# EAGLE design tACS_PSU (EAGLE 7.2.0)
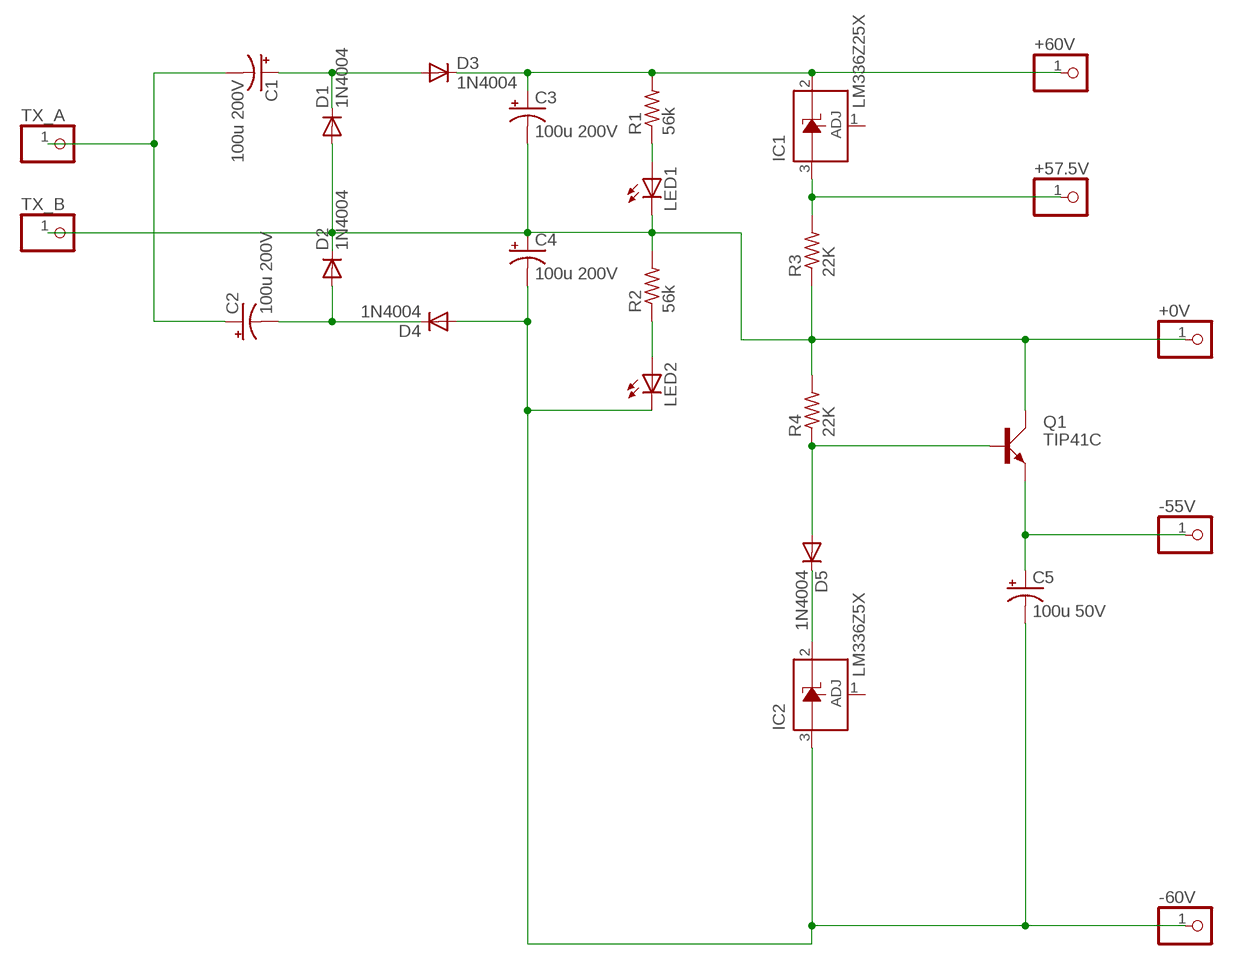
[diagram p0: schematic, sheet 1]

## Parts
+0V  PINHD-1X1  [1X01]
+57.5V  PINHD-1X1  [1X01]
+60V  PINHD-1X1  [1X01]
-55V  PINHD-1X1  [1X01]
-60V  PINHD-1X1  [1X01]
C1  100u 200V  CPOL-USE7.5-18  [E7,5-18]
C2  100u 200V  CPOL-USE7.5-18  [E7,5-18]
C3  100u 200V  CPOL-USE7.5-18  [E7,5-18]
C4  100u 200V  CPOL-USE7.5-18  [E7,5-18]
C5  100u 50V  CPOL-USE3.5-10  [E3,5-10]
D1  1N4004  [DO41-10]
D2  1N4004  [DO41-10]
D3  1N4004  [DO41-10]
D4  1N4004  [DO41-10]
D5  1N4004  [DO41-10]
IC1  LM336Z25X  LM336LP  [TO92]
IC2  LM336Z5X  LM336LP  [TO92]
LED1  LED5MM  [LED5MM]
LED2  LED5MM  [LED5MM]
Q1  TIP41C  [TO220AV]
R1  56k  R-US_0207/10  [0207/10]
R2  56k  R-US_0207/10  [0207/10]
R3  22K  R-US_0207/10  [0207/10]
R4  22K  R-US_0207/10  [0207/10]
TX_A  PINHD-1X1  [1X01]
TX_B  PINHD-1X1  [1X01]

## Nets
N$1: C1.- C2.+ TX_A.1
N$2: +0V.1 C3.- C4.+ D1.A D2.C LED1.K(C) Q1.C R2.2 R3.1 R4.2 TX_B.1
N$3: C2.- D2.A D4.C
N$4: C1.+ D1.C D3.A
N$5: +60V.1 C3.+ D3.C IC1.2(C) R1.2
N$6: -55V.1 C5.+ Q1.E
N$7: -60V.1 C4.- C5.- D4.A IC2.3(A) LED2.K(C)
N$8: LED1.A R1.1
N$10: LED2.A R2.1
N$11: +57.5V.1 IC1.3(A) R3.2
N$12: D5.A Q1.B R4.1
N$13: D5.C IC2.2(C)
Unconnected: IC1.1(ADJ) IC2.1(ADJ)

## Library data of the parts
+0V +57.5V +60V -55V -60V TX_A TX_B = pinhead:PINHD-1X1: PIN HEADER
C1-C5 = rcl:CPOL-US: POLARIZED CAPACITOR, American symbol
D1-D5 = diode:1N4004: DIODE
IC1 IC2 = linear:LM336: 2.5-V INTEGRATED REFERENCE CIRCUITS LM236 Source: http://focus.ti.com/lit/ds/symlink/lm336-2.5.pdf
LED1 LED2 = led:LED: LED
Q1 = transistor-power:TIP41C: NPN TRANSISTOR
R1-R4 = rcl:R-US_: RESISTOR, American symbol

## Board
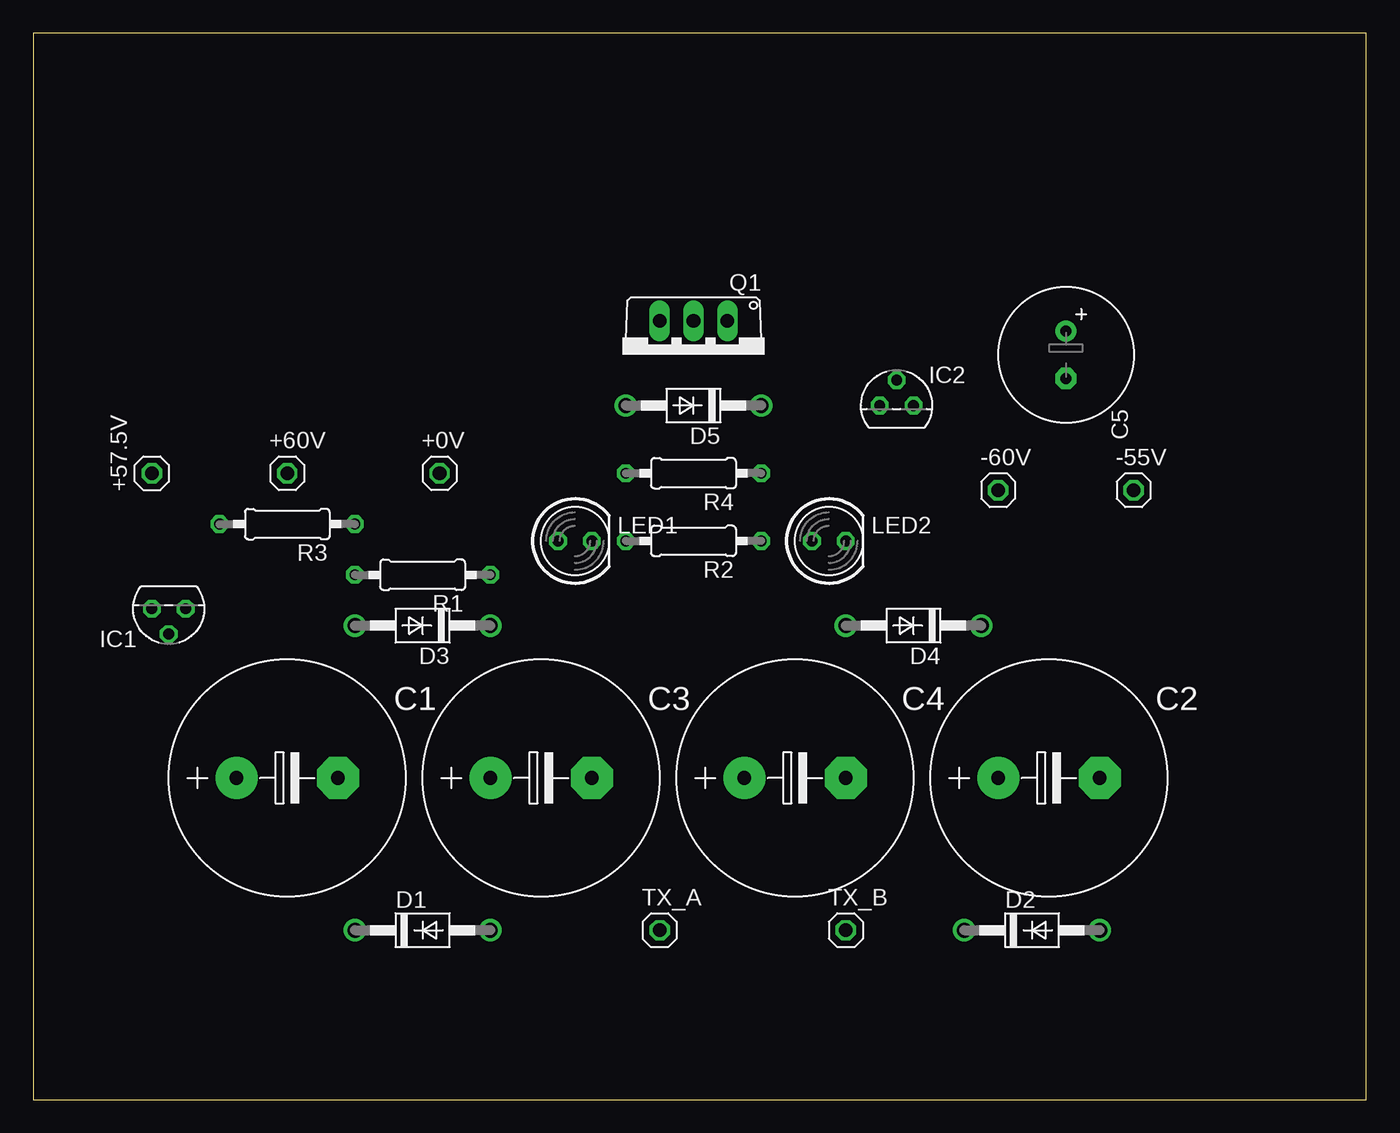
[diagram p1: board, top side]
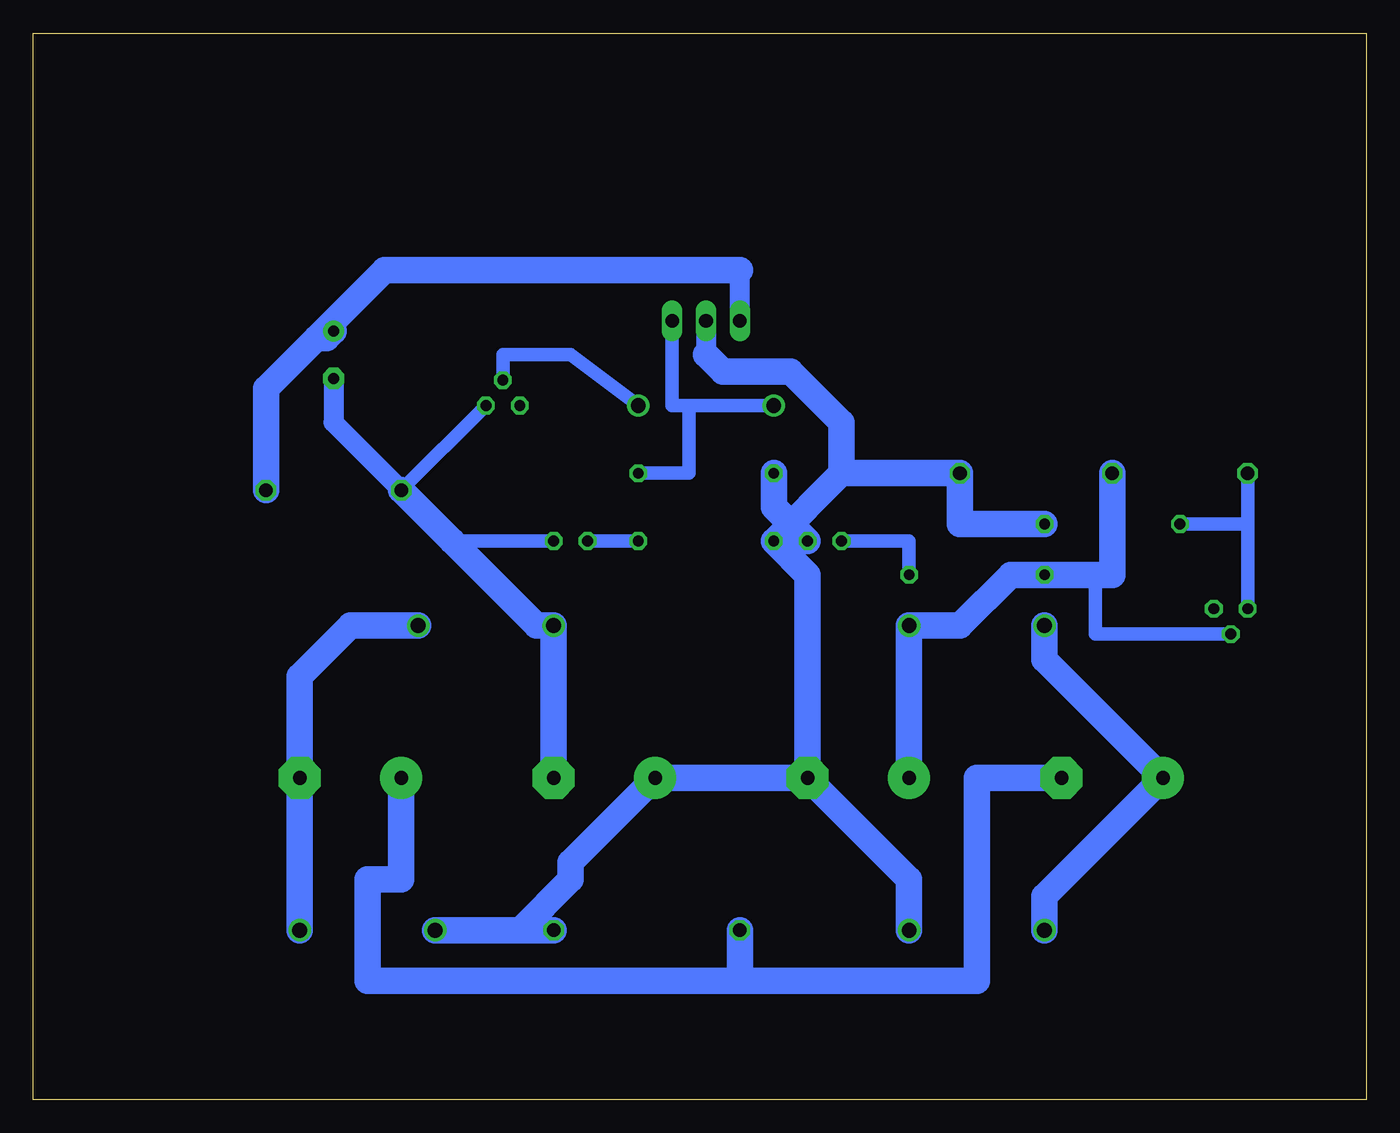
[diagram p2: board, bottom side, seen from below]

Size 100 x 80 mm. Coordinates in mm from the lower left corner, seen from the top.
Outline: 0,0 100,0 100,80 0,80 0,0
Copper layers (1*16): Top 0.035mm / dielectric 1.5mm / Bottom 0.035mm
Design rules "default": minimum track width 10mil, minimum drill 24mil, track to track 8mil, track to pad 8mil, pad to pad 8mil, via to via 8mil, smd to smd 8mil, copper to edge 40mil, drill to drill 8mil, minimum pad ring 10mil, minimum via ring 8mil, stop-mask expansion 4mil, vias tented up to drill 0mil, thermal gap 10mil

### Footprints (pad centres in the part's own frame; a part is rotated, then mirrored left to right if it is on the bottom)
1X01 = drill 1.016 octagon: 1 0,0
E7,5-18 = drill 1.016 pad 3.15: + -3.81,0 | drill 1.016 pad 3.15 octagon: - 3.81,0
E3,5-10 = drill 0.813 pad 1.6: + -1.778,0 | drill 0.813 pad 1.6 octagon: - 1.778,0
DO41-10 = drill 1.118: A 5.08,0; C -5.08,0
TO92 = drill 0.813 octagon: 1 -1.27,0; 2 0,1.905; 3 1.27,0
LED5MM = drill 0.813 octagon: A -1.27,0; K 1.27,0
TO220AV = drill 1.016 long: B -2.54,-2.54; C 0,-2.54; E 2.54,-2.54
0207/10 = drill 0.813 octagon: 1 -5.08,0; 2 5.08,0

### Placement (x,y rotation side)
+0V  30.48,46.99 0 top
+57.5V  8.89,46.99 90 top
+60V  19.05,46.99 0 top
-55V  82.55,45.72 0 top
-60V  72.39,45.72 0 top
C1  19.05,24.13 0 top
C2  76.2,24.13 0 top
C3  38.1,24.13 0 top
C4  57.15,24.13 0 top
C5  77.47,55.88 270 top
D1  29.21,12.7 0 top
D2  74.93,12.7 0 top
D3  29.21,35.56 180 top
D4  66.04,35.56 180 top
D5  49.53,52.07 180 top
IC1  10.16,36.83 180 top
IC2  64.77,52.07 0 top
LED1  40.64,41.91 0 top
LED2  59.69,41.91 0 top
Q1  49.53,55.88 180 top
R1  29.21,39.37 180 top
R2  49.53,41.91 180 top
R3  19.05,43.18 180 top
R4  49.53,46.99 180 top
TX_A  46.99,12.7 0 top
TX_B  60.96,12.7 0 top

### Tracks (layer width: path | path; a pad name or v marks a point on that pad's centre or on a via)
N$1
  Bottom 2: C1.- 29.21,24.13 29.21,8.89 46.99,8.89 | 46.99,8.89 TX_A.1 | C2.+ 72.39,16.51 74.93,16.51 74.93,8.89 46.99,8.89
N$2
  Bottom 1.5: Q1.C 49.53,55.88
  Bottom 2: C3.- C4.+ 59.69,17.78 59.69,16.51 63.5,12.7 | D1.A 34.29,16.51 C3.- | C3.- 41.91,39.37 R2.2 | R2.2 LED1.K 44.45,44.45 R4.2 | 39.37,46.99 +0V.1 30.48,43.18 R3.1 | 39.37,46.99 R2.2 | 49.53,55.88 48.26,54.61 43.18,54.61 39.37,50.8 39.37,46.99 | TX_B.1 63.5,12.7 | 63.5,12.7 D2.C
N$3
  Bottom 2: D2.A C2.- 80.01,31.75 76.2,35.56 D4.C
N$4
  Bottom 2: D3.A 24.13,33.02 C1.+ 24.13,15.24 D1.C
N$5
  Bottom 1: IC1.2 20.32,34.92 20.32,39.37 26.67,39.37
  Bottom 2: C3.+ D3.C 30.48,35.56 26.67,39.37 R1.2 19.05,39.37 +60V.1
N$6
  Bottom 1.5: Q1.E 46.99,62.23
  Bottom 2: -55V.1 82.55,53.34 78.74,57.15 | 78.74,57.15 77.98,57.15 C5.+ | 46.99,62.23 73.66,62.23 78.74,57.15
N$7
  Bottom 1: -60V.1 IC2.3 | LED2.K 68.58,41.91
  Bottom 1.5: C5.- 77.47,50.8 -60V.1
  Bottom 2: C4.- D4.A 62.23,35.56 68.58,41.91 -60V.1
N$8
  Bottom 1: R1.1 34.29,41.91 LED1.A
N$10
  Bottom 1: LED2.A R2.1
N$11
  Bottom 1: IC1.3 8.89,43.18 | R3.2 8.89,43.18 | 8.89,43.18 +57.5V.1
N$12
  Bottom 1: D5.A 50.8,52.07 | 50.8,52.07 52.07,52.07 Q1.B | R4.1 50.8,46.99 50.8,52.07
N$13
  Bottom 1: D5.C 59.69,55.88 64.77,55.88 IC2.2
